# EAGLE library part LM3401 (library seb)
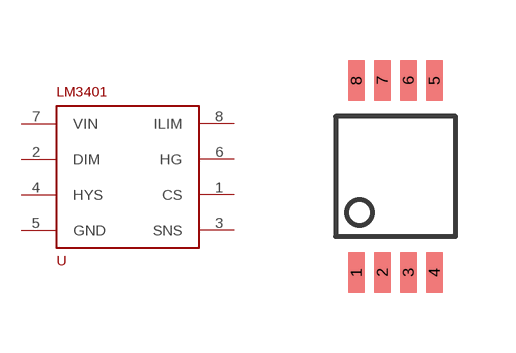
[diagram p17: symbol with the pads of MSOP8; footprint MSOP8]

Designator prefix -

## LM3401  [MSOP8]
1  CS
2  DIM
3  SNS
4  HYS
5  GND
6  HG
7  VIN
8  ILIM

## Footprint MSOP8 (pad centres in mm)
smd 0.41 x 1.02: 1 -0.975,-2.4; 2 -0.325,-2.4; 3 0.325,-2.4; 4 0.975,-2.4; 5 0.975,2.4; 6 0.325,2.4; 7 -0.325,2.4; 8 -0.975,2.4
